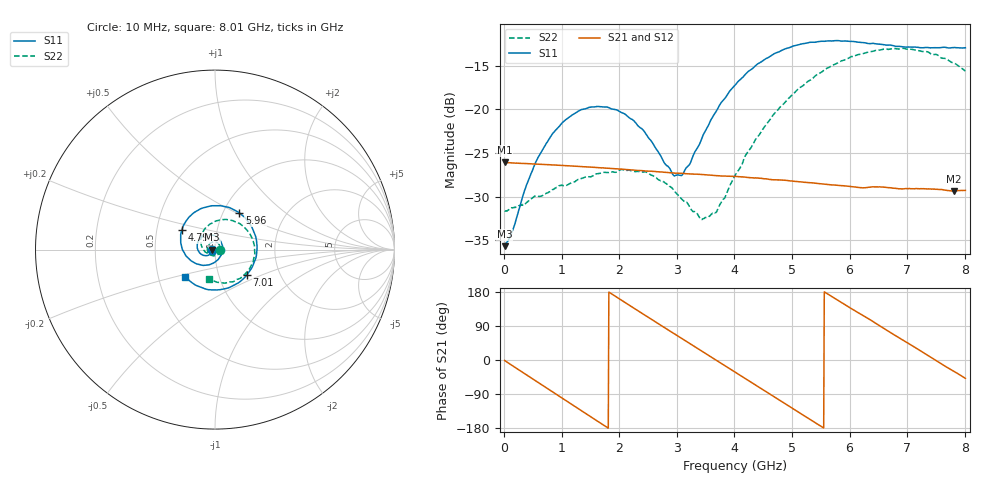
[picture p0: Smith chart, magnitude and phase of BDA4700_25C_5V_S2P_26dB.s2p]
!Agilent Technologies,E5071B,MY42404982,A.09.10
!Date: Mon Oct 20 13:39:35 2025
!Data & Calibration Information:
!Freq	S11:SOLT2(ON)	S21:SOLT2(ON)	S12:SOLT2(ON)	S22:SOLT2(ON)
# Hz S RI R 50
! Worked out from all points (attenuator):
!   801 points, 10 MHz to 8.01 GHz, reference 50 ohm
!   highest |S21| = -26.07 dB at 10 MHz (marker M1); lowest = -29.3 dB at 7.81 GHz (marker M2)
!   lowest |S11| = -35.7 dB at 10 MHz (marker M3), VSWR 1.03, Z = 48.4 - j0.111 ohm
!   |S11| at or under -10 dB: start of sweep to end of sweep
!   |S22| runs from -32.6 to -13.0 dB; largest |S21 - S12| = 0.00043
!   S11 on the Smith chart (normalised r, x): 10 MHz: 0.97, -0.00; 4.79 GHz: 0.67, +0.15; 5.96 GHz: 1.19, +0.52; 7.01 GHz: 1.36, -0.41; 8.01 GHz: 0.69, -0.22
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1e7  -0.0165 -0.00115  0.0497 -0.00104  0.0497 -0.00112  0.0262 -0.000811
1.4e8  -0.0177 -0.00936  0.0478 -0.0123  0.0478 -0.0123  0.0265 -0.00679
3.8e8  -0.0265 -0.0245  0.0383 -0.0304  0.0383 -0.0305  0.0213 -0.0197
6.2e8  -0.0436 -0.0336  0.0225 -0.0429  0.0225 -0.043  0.0115 -0.0296
1.01e9  -0.0804 -0.0232  -0.00913 -0.0469  -0.00917 -0.0469  -0.0153 -0.0335
1.35e9  -0.0993 0.00986  -0.033 -0.0335  -0.033 -0.0335  -0.0361 -0.0177
2.08e9  -0.0467 0.0823  -0.0407 0.02  -0.0407 0.02  -0.0297 0.0337
2.68e9  0.0309 0.0478  -0.00438 0.0437  -0.00437 0.0437  0.013 0.0374
2.94e9  0.0414 0.00747  0.0142 0.0408  0.0144 0.0408  0.0252 0.024
3.09e9  0.038 -0.0179  0.0239 0.0358  0.0237 0.0358  0.028 0.0122
3.41e9  0.00481 -0.0649  0.0382 0.0184  0.0383 0.0183  0.0205 -0.0119
3.54e9  -0.0165 -0.0781  0.041 0.00962  0.0411 0.00954  0.0129 -0.0205
3.7e9  -0.0494 -0.0863  0.0417 -0.00155  0.0417 -0.00163  -0.000704 -0.0264
4.01e9  -0.1165 -0.0725  0.0351 -0.0218  0.0352 -0.0217  -0.0325 -0.026
4.79e9  -0.1845 0.1094  -0.0114 -0.0377  -0.0112 -0.0378  -0.0788 0.0657
5.35e9  -0.0665 0.2324  -0.0357 -0.0128  -0.0357 -0.0128  -0.0153 0.1481
5.96e9  0.1364 0.2039  -0.0287 0.0223  -0.0288 0.0222  0.1224 0.1517
6.68e9  0.2309 -0.0305  0.00915 0.0345  0.0092 0.0345  0.2204 -8.99e-05
7.01e9  0.1767 -0.1424  0.0249 0.0249  0.025 0.0247  0.2017 -0.0889
7.42e9  0.0426 -0.2207  0.0348 0.00383  0.0348 0.00376  0.1225 -0.1661
7.81e9  -0.1046 -0.1994  0.0296 -0.017  0.0296 -0.0171  0.017 -0.183
8.01e9  -0.1646 -0.1532  0.0228 -0.0258  0.0228 -0.0257  -0.0314 -0.1622
